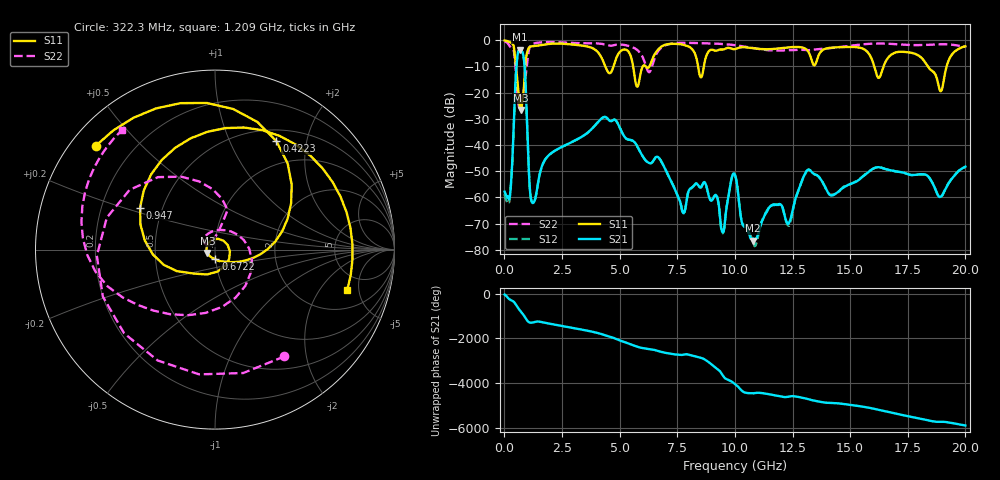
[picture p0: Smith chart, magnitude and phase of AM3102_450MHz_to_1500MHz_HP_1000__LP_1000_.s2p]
!Agilent Technologies,E8364B,MY43040894,A.07.50.67
!Agilent E8364B: A.07.50.67
!Date: Thursday, January 11, 2018 05:58:26
!Correction: S11(Full 2 Port(1,2))
!S21(Full 2 Port(1,2))
!S12(Full 2 Port(1,2))
!S22(Full 2 Port(1,2))
!S2P File: Measurements: S11, S21, S12, S22:
# Hz S  dB  R 50
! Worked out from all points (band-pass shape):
!   1601 points, 10 MHz to 20 GHz, reference 50 ohm
!   highest |S21| = -3.60 dB at 672.2 MHz (marker M1); lowest = -76.5 dB at 10.77 GHz (marker M2)
!   |S21| within 3 dB of the highest: 557.7 MHz to 839.5 MHz (281.8 MHz wide, 40.3 % of centre)
!   lowest |S11| = -26.7 dB at 709.6 MHz (marker M3), VSWR 1.10, Z = 45.9 - j1.79 ohm
!   |S11| at or under -10 dB: 503.3 MHz to 901.9 MHz (398.6 MHz wide, 56.7 % of centre); 5.586 GHz to 6.002 GHz (415.8 MHz wide, 7.18 % of centre); 18.37 GHz to 19.18 GHz (816.7 MHz wide, 4.35 % of centre)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
!   |S22| runs from -25.6 to -0.4 dB; largest |S21 - S12| = 0.0016
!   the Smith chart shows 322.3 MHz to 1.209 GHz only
!   S11 on the Smith chart (normalised r, x): 322.3 MHz: 0.07, +0.37; 422.3 MHz: 0.65, +1.52; 672.2 MHz: 1.00, -0.11; 947 MHz: 0.37, +0.23; 1.209 GHz: 3.38, -3.76
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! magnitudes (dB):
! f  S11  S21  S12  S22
! 10 MHz  -0.1  -57.8  -58.6  -0.4
! 322.3 MHz  -1.1  -49.8  -50.2  -3.0
! 422.3 MHz  -3.2  -28.1  -28.1  -4.7
! 672.2 MHz  -25.5  -3.6  -3.6  -25.6
! 709.6 MHz  -26.7  -3.7  -3.7  -24.4
! 947 MHz  -6.4  -22.6  -22.5  -11.6
! 1.209 GHz  -2.3  -61.9  -62.0  -1.5
! 3.346 GHz  -2.0  -36.9  -36.9  -1.1
! 5.307 GHz  -3.7  -37.7  -37.7  -2.0
! 5.77 GHz  -17.7  -40.6  -40.6  -3.8
! 6.682 GHz  -3.4  -44.7  -44.7  -4.0
! 7.744 GHz  -1.7  -65.7  -66.1  -1.0
! 8.681 GHz  -8.6  -54.1  -54.4  -1.1
! 9.468 GHz  -3.5  -73.2  -73.7  -1.4
! 10.01 GHz  -3.4  -51.5  -51.4  -1.9
! 10.77 GHz  -3.0  -76.5  -76.2  -2.9
! 11.62 GHz  -3.3  -62.9  -63.1  -3.9
! 12.35 GHz  -2.7  -69.6  -70.9  -3.8
! 13.34 GHz  -8.0  -50.4  -50.4  -3.7
! 16.68 GHz  -6.4  -49.5  -49.5  -1.3
! 18.93 GHz  -19.4  -59.7  -60.0  -1.5
! 20 GHz  -2.3  -48.2  -48.4  -2.5
